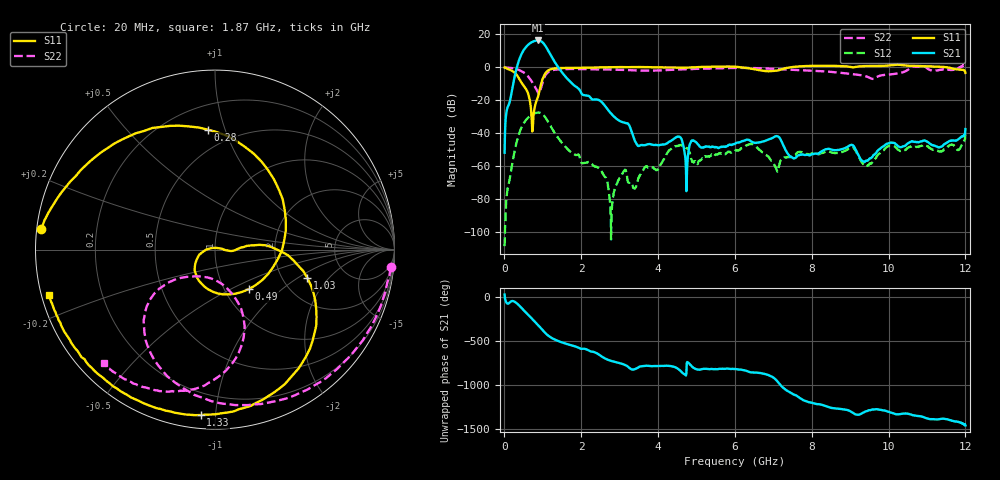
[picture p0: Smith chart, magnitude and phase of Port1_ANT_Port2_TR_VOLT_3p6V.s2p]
! Created Mon Aug 25 11:24:29 2025
# hz S ma R 50
! 2 Port Network Data from SP1.SP block
! freq  magS11  angS11  magS21  angS21  magS12  angS12  magS22  angS22
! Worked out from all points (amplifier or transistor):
!   1200 points, 10 MHz to 12 GHz, reference 50 ohm
!   highest |S21| = 16.3 dB at 870 MHz (marker M1)
!   |S21| within 3 dB of that: 604.6 MHz to 1.062 GHz (457.9 MHz wide, 54.9 % of centre)
!   unconditionally stable (mu >= 1): start of sweep to 2.671 GHz; 3.949 GHz to 4.98 GHz; 6.17 GHz to 7.451 GHz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
!   at 2.01 GHz: K = 42.20, MAG = 1.8 dB, |S12| = -58.0 dB
!   at 6.01 GHz: K = -235.64, MSG = 2.1 dB, |S12| = -50.6 dB
!   at 12 GHz: K = -1736.36, MSG = 1.5 dB, |S12| = -40.6 dB
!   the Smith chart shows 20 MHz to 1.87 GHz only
!   S11 on the Smith chart (normalised r, x): 20 MHz: 0.01, +0.06; 280 MHz: 0.36, +0.87; 490 MHz: 1.30, -0.62; 1.03 GHz: 2.73, -1.22; 1.33 GHz: 0.07, -0.91; 1.87 GHz: 0.02, -0.13
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1e7  0.9818 176.4  0.002563 28.6  3.713e-06 -177.7  0.9899 -3.2
2e7  0.9744 173.1  0.01017 -15.0  1.161e-05 -124.3  0.9851 -5.8
2.8e8  0.6696 93.4  0.5842 -56.0  0.003234 157.2  0.9024 -71.1
3.8e8  0.4704 36.7  1.572 -92.4  0.009145 118.4  0.8323 -93.9
4.9e8  0.2907 -49.1  3.085 -142.7  0.01846 67.7  0.7164 -116.5
5.8e8  0.2043 -111.4  4.3 176.4  0.02626 27.3  0.5891 -132.1
6.6e8  0.1069 -155.2  5.244 140.6  0.03252 -7.8  0.4597 -142.3
7.7e8  0.04296 4.4  6.168 91.4  0.03902 -55.9  0.2967 -143.9
8.7e8  0.1193 0.3  6.512 45.7  0.04203 -100.2  0.1788 -123.5
9.5e8  0.2795 5.0  6.237 6.7  0.04096 -138.2  0.2213 -73.3
1.03e9  0.5392 -17.1  5.202 -33.0  0.0347 -176.8  0.4566 -68.8
1.17e9  0.8313 -60.1  2.825 -88.2  0.01938 130.3  0.7448 -92.9
1.33e9  0.9251 -94.9  1.359 -127.7  0.009466 94.4  0.847 -111.4
1.87e9  0.9574 -164.8  0.2547 153.8  0.002155 46.2  0.8851 -134.6
2.01e9  0.9604 -174.1  0.1598 129.5  0.001257 27.4  0.8848 -136.9
2.79e9  1.003 174.1  0.03827 -9.2  2.535e-05 137.0  0.8543 -148.7
4.01e9  0.995 177.2  0.004289 -66.3  0.0008062 54.3  0.8009 142.0
6.01e9  1.035 145.8  0.004795 -100.3  0.002953 -42.6  0.9523 125.0
8.01e9  1.101 71.1  0.002318 -126.0  0.002438 -97.8  0.7875 141.6
1.001e10  1.136 -176.4  0.004976 131.2  0.004049 130.3  0.6015 103.7
1.099e10  1.068 -137.2  0.005659 57.5  0.004131 46.9  0.9597 66.3
1.2e10  0.6757 -71.4  0.01329 -24.2  0.009341 -51.6  1.339 -171.9
